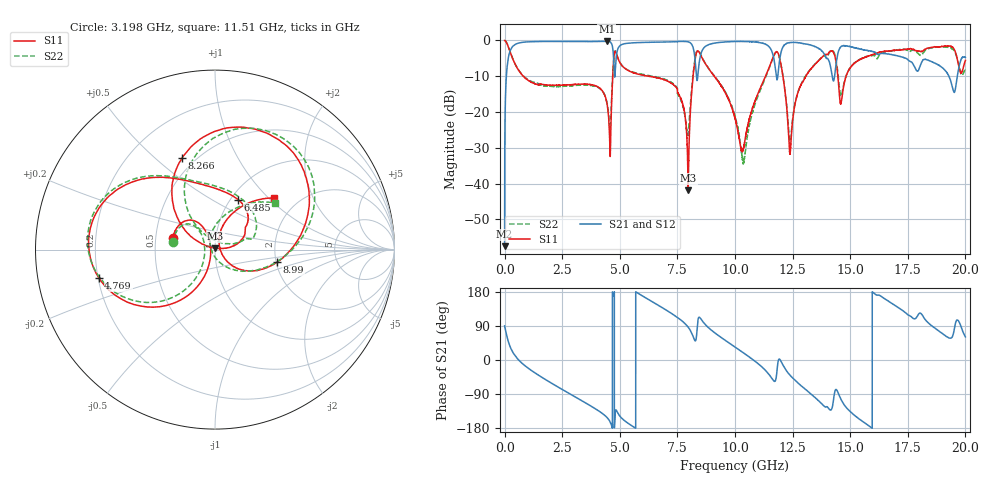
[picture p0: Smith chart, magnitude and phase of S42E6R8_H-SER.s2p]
!{S42E6R8}
!Johanson Technology Inc.
!www.johansontechnology.com
!Test Board Conditions:
!Substrate Type  RO4350B
!Substrate Thickness  50 mil
!Substrate Dk  3.66
!TL Type: GCPW
!TL Trace Width  60 mil
!TL Gap  10 mil
!Electrode orientation  Horizontal
!DUT TOPOLOGY	SERIES
!Mounting Pad LxW  14x55 mil
! Created Wed Nov 25 21:49:42 2020
# khz S ma R 50
! 2 Port Network Data from SP1.SP block
! freq  magS11  angS11  magS21  angS21  magS12  angS12  magS22  angS22
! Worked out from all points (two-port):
!   20001 points, 300 kHz to 20 GHz, reference 50 ohm
!   highest |S21| = -0.23 dB at 4.432 GHz (marker M1); lowest = -57.5 dB at 300 kHz (marker M2)
!   |S21| within 3 dB of the highest: 223.9 MHz to 4.712 GHz (4.488 GHz wide, 182 % of centre); 4.878 GHz to 8.225 GHz (3.347 GHz wide, 51.1 % of centre)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
!   lowest |S11| = -41.9 dB at 7.968 GHz (marker M3), VSWR 1.02, Z = 50.1 + j0.799 ohm
!   |S11| at or under -10 dB: 812.8 MHz to 4.693 GHz (3.88 GHz wide, 141 % of centre); 6.252 GHz to 8.18 GHz (1.927 GHz wide, 26.7 % of centre); 9.102 GHz to 11.32 GHz (2.221 GHz wide, 21.7 % of centre)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
!   |S22| runs from -34.6 to 0.0 dB; largest |S21 - S12| = 0.021
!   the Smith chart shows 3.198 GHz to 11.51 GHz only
!   S11 on the Smith chart (normalised r, x): 3.198 GHz: 0.61, +0.08; 4.769 GHz: 0.20, -0.11; 6.485 GHz: 1.08, +0.66; 8.266 GHz: 0.43, +0.62; 8.99 GHz: 2.02, -0.32; 11.51 GHz: 1.52, +1.08
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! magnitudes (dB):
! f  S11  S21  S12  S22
! 300 kHz  0.0  -57.5  -57.6  0.0
! 111.3 MHz  -0.9  -7.2  -7.2  -0.9
! 305.3 MHz  -4.3  -2.1  -2.1  -4.3
! 3.198 GHz  -12.2  -0.3  -0.3  -12.5
! 3.334 GHz  -12.2  -0.3  -0.3  -12.5
! 4.432 GHz  -17.2  -0.2  -0.2  -17.0
! 4.579 GHz  -32.3  -0.4  -0.4  -24.8
! 4.769 GHz  -3.5  -9.8  -9.8  -3.4
! 6.485 GHz  -10.3  -0.5  -0.5  -10.1
! 6.667 GHz  -10.5  -0.5  -0.5  -10.3
! 7.968 GHz  -41.9  -0.4  -0.4  -25.8
! 8.266 GHz  -5.3  -5.3  -5.3  -5.0
! 8.99 GHz  -9.1  -0.9  -0.9  -8.9
! 10 GHz  -21.7  -0.3  -0.3  -21.1
! 10.38 GHz  -29.6  -0.3  -0.3  -34.0
! 11.51 GHz  -7.2  -1.9  -2.0  -7.4
! 11.92 GHz  -4.5  -6.1  -6.1  -4.6
! 12.39 GHz  -31.3  -0.6  -0.6  -28.6
! 13.33 GHz  -7.7  -1.4  -1.4  -7.6
! 14.61 GHz  -17.3  -1.7  -1.7  -15.4
! 16.67 GHz  -3.0  -3.8  -4.0  -3.0
! 20 GHz  -5.6  -4.8  -4.7  -8.3
